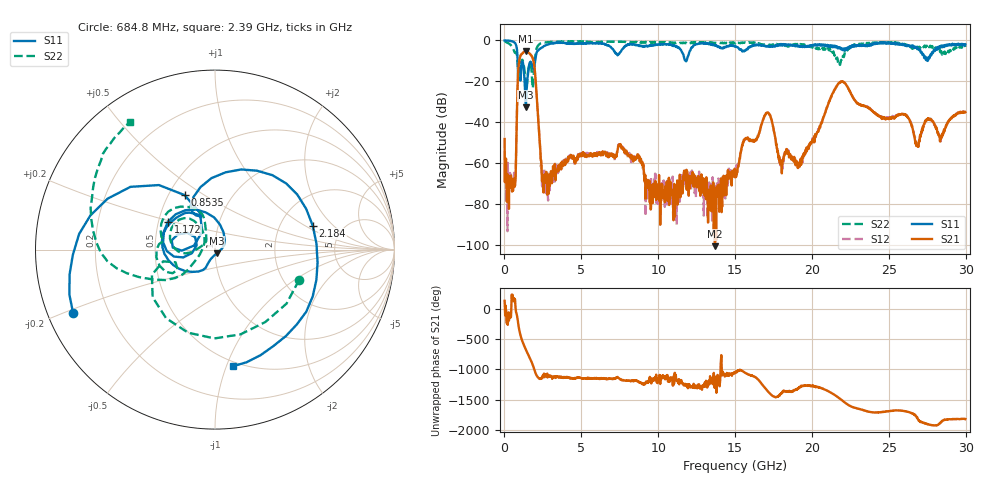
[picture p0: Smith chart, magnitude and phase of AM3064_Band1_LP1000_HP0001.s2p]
# Hz S DB R 50.0
!freq dBS11 angS11 dBS21 angS21 dBS12 angS12 dBS22 angS22
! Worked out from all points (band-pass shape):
!   1600 points, 10 MHz to 29.98 GHz, reference 50 ohm
!   highest |S21| = -5.22 dB at 1.397 GHz (marker M1); lowest = -100.4 dB at 13.69 GHz (marker M2)
!   |S21| within 3 dB of the highest: 1.013 GHz to 1.811 GHz (798.2 MHz wide, 56.5 % of centre)
!   lowest |S11| = -32.7 dB at 1.397 GHz (marker M3), VSWR 1.05, Z = 50.9 - j2.16 ohm
!   |S11| at or under -10 dB: 857.4 MHz to 1.997 GHz (1.139 GHz wide, 79.8 % of centre); 11.78536 GHz to 11.83828 GHz (52.92 MHz wide, 0.448 % of centre); 27.52527 GHz to 27.52945 GHz (4.185 MHz wide, 0.0152 % of centre)
!   |S22| runs from -23.6 to -0.4 dB; largest |S21 - S12| = 0.0063
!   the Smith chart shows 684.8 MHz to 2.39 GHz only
!   S11 on the Smith chart (normalised r, x): 684.8 MHz: 0.08, -0.21; 853.5 MHz: 0.60, +0.42; 1.172 GHz: 0.56, +0.19; 2.184 GHz: 3.05, +1.18; 2.39 GHz: 0.46, -1.06
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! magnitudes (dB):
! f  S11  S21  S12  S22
! 10 MHz  0.0  -48.1  -54.2  -0.4
! 291.2 MHz  -0.2  -82.2  -72.3  -1.6
! 684.8 MHz  -1.3  -70.7  -70.9  -6.1
! 853.5 MHz  -9.2  -22.5  -22.4  -10.6
! 1.172 GHz  -10.3  -6.4  -6.3  -9.5
! 1.397 GHz  -32.7  -5.2  -5.2  -22.4
! 1.866 GHz  -13.6  -9.4  -9.4  -21.1
! 2.184 GHz  -5.0  -36.8  -36.7  -2.6
! 2.39 GHz  -3.6  -59.2  -58.7  -1.4
! 2.803 GHz  -2.0  -65.5  -66.7  -0.9
! 5.015 GHz  -1.4  -56.2  -54.9  -0.8
! 7.564 GHz  -5.6  -51.7  -51.2  -0.6
! 10 GHz  -2.0  -70.3  -74.5  -0.9
! 13.69 GHz  -2.3  -100.4  -71.0  -1.2
! 15 GHz  -2.8  -66.8  -66.0  -1.5
! 17.07 GHz  -2.7  -35.3  -35.3  -2.3
! 17.99 GHz  -2.4  -59.7  -58.8  -2.4
! 19.99 GHz  -2.8  -49.2  -49.1  -3.1
! 21.88 GHz  -4.0  -20.4  -20.2  -9.8
! 25 GHz  -1.0  -38.4  -37.5  -1.1
! 26.85 GHz  -4.3  -51.2  -50.9  -3.1
! 29.98 GHz  -1.9  -35.0  -34.9  -3.2
